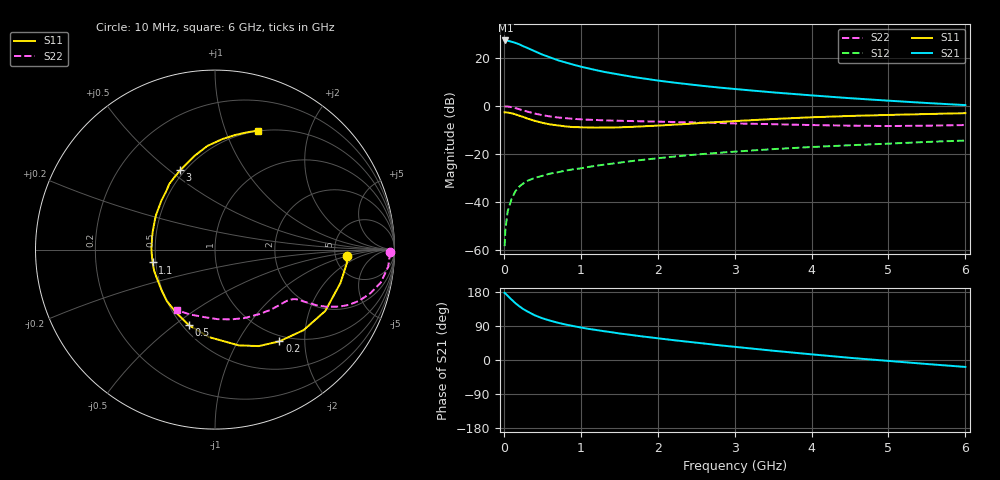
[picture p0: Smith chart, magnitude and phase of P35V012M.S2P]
! SIEMENS Small Signal Semiconductors
! BFP181
! Si NPN RF Bipolar Junction Transistor in SOT143
! VCE = 5 V  IC = 12 mA
! Common Emitter S-Parameters:  March  1996
# GHz  S  MA  R  50
!  f  S11  S21  S12  S22
! GHz  MAG  ANG  MAG  ANG  MAG  ANG  MAG  ANG
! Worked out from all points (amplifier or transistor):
!   36 points, 10 MHz to 6 GHz, reference 50 ohm
!   highest |S21| = 27.2 dB at 20 MHz (marker M1)
!   |S21| within 3 dB of that: start of sweep to 297.3 MHz
!   unconditionally stable (mu >= 1): 1.127 GHz to end of sweep
!   at 250 MHz: K = 0.36, MSG = 28.6 dB, |S12| = -32.4 dB
!   at 1.4 GHz: K = 1.08, MAG = 17.1 dB, |S12| = -24.1 dB
!   at 6 GHz: K = 1.00, MAG = 7.2 dB, |S12| = -14.4 dB
!   S11 on the Smith chart (normalised r, x): 10 MHz: 6.33, -1.05; 200 MHz: 0.91, -1.52; 500 MHz: 0.54, -0.56; 1.1 GHz: 0.48, -0.08; 3 GHz: 0.47, +0.55; 6 GHz: 0.49, +1.31
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0.01  0.7338 -3.0  22.93 177.3  0.0012 84.8  0.9776 -0.9
0.02  0.7385 -5.9  23.03 175.7  0.0026 83.0  0.9738 -2.2
0.05  0.7233 -14.9  22.73 169.3  0.0064 86.3  0.9692 -5.7
0.1  0.7032 -29.1  21.64 159.5  0.0115 74.5  0.9421 -11.2
0.15  0.6669 -42.3  20.51 150.0  0.0167 69.8  0.8995 -15.7
0.2  0.6247 -54.9  19.16 141.9  0.0208 65.2  0.8531 -19.5
0.25  0.5904 -65.6  17.54 134.7  0.0241 62.2  0.8073 -22.4
0.3  0.5497 -76.1  16.23 128.8  0.0273 59.1  0.7654 -24.5
0.4  0.4887 -93.9  13.77 118.1  0.0316 54.8  0.6939 -27.3
0.5  0.4448 -109.3  11.71 110.2  0.035 52.1  0.641 -28.8
0.6  0.4123 -121.8  10.24 103.9  0.0389 51.3  0.6031 -29.6
0.7  0.3926 -133.1  8.949 98.5  0.0414 51.1  0.5746 -30.3
0.9  0.3623 -151.9  7.249 89.7  0.0478 50.8  0.5381 -31.1
1.1  0.355 -168.4  6.031 82.2  0.0536 50.9  0.5154 -32.4
1.3  0.3545 179.0  5.124 76.1  0.0597 50.2  0.5008 -34.1
1.6  0.3627 162.3  4.215 67.6  0.0688 50.1  0.4859 -36.9
2.2  0.4055 137.2  3.07 52.5  0.0877 47.6  0.4622 -44.7
3  0.4825 113.7  2.247 34.8  0.1115 42.3  0.4313 -57.3
3.5  0.5328 102.7  1.91 24.5  0.1259 38.8  0.4156 -66.6
4.5  0.6171 86.2  1.446 5.7  0.1515 30.8  0.3875 -88.1
5.5  0.6765 74.9  1.148 -10.6  0.1775 23.7  0.3871 -110.9
6  0.7057 70.0  1.038 -18.3  0.1902 19.5  0.3992 -122.5
